FUNCTION_BLOCK Axis_IO
VAR_INPUT
	snHome:			BOOL;(*原点*)
	snLimitP:		BOOL;(*正限*)
	snLimitN:		BOOL;(*负限*)
	btManualJogF:	BOOL;(*点动按钮正*)
	btManualJogB:	BOOL;(*点动按钮负*)
	DriverDI:		ServoDriver_DI;(*伺服驱动器的输入*)
END_VAR

;

END_FUNCTION_BLOCK
